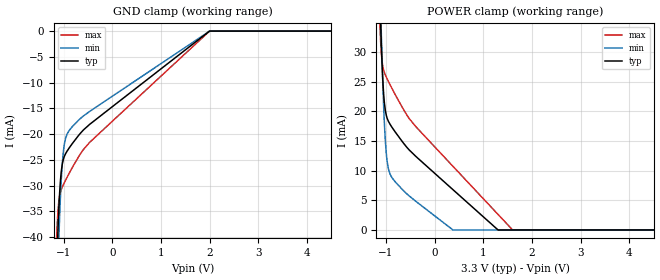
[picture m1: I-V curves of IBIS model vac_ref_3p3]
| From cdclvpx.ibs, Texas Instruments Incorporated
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|Pulldown resistor value available only for typ corner, user may use the same
|value across min and max corners as well
|   Vac_ref_3p3 Model   |
[Model]   vac_ref_3p3
Model_type   Terminator
| Signals   VAC_REF
| variable   typ   min   max
C_comp   0.151pF   0.149pF   0.158pF
| Where nom  PVT is Nominal Process, 3.3V, 40C
|   Fast PVT is Strong Process,  3.6V, -40C
|   Slow PVT is Weak Process,   2.375V,100C
| Junction Temperature (Ambient temp is 25C typ, 85C min, -40C max)
[Temperature Range]   40C   100C   -40C
[Voltage range]   3.3V   2.375V   3.6V
[GND Clamp]
|   Voltage   I(typ)   I(min)   I(max)
-3.3V     -1.088A    -1.091A    -1.088A
-1.146V   -47.72mA   -55.84mA   -40.84mA
-1.114V   -38.55mA   -45.35mA   -34.88mA
-1.097V   -34.54mA   -40.29mA   -33.06mA
-1.089V   -33.03mA   -38.25mA   -32.5mA
-1.05V    -27.53mA   -29.4mA    -30.85mA
-1.006V   -24.96mA   -23.55mA   -29.86mA
-956.2mV  -23.77mA   -20.75mA   -28.92mA
-874.5mV  -22.56mA   -19.17mA   -27.44mA
-468.3mV  -18.15mA   -15.63mA   -21.65mA
1.999V    -4.541uA   -4.591uA   -5.065uA
6.598V    0A         0A         0A
[POWER Clamp]
|   Voltage   I(typ)   I(min)   I(max)
-3.3V     1.09A      1.087A     1.093A
-1.122V   37.89mA    40.65mA    33.58mA
-1.104V   33.15mA    35.14mA    30.75mA
-1.065V   24.97mA    24.2mA     27.52mA
-1.015V   20.19mA    15.11mA    26.16mA
-973.5mV  18.75mA    11.35mA    25.42mA
-916.6mV  17.81mA    9.411mA    24.49mA
-530mV    13.54mA    5.784mA    18.85mA
375.3mV   6.793mA    0A         10.73mA
1.301V    0A         0A         2.617mA
1.601V    0A         0A         4.06pA
6.598V    0A         0A         0A
